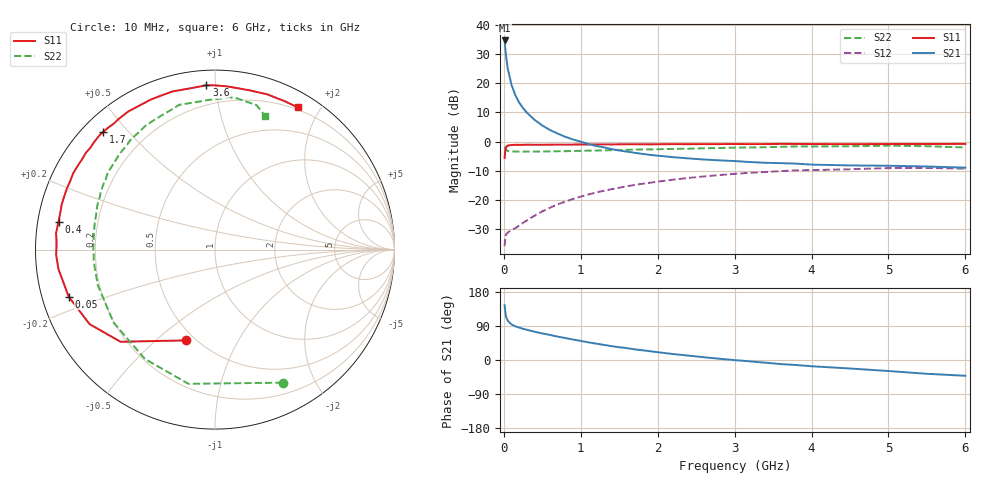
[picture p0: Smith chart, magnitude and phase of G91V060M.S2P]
! SIEMENS Small Signal Semiconductors
! BFG235
! Si NPN RF Bipolar Junction Transistor in SOT223
! VCE = 1 V  IC = 60 mA
! Common Emitter S-Parameters:  July  1994
# GHz  S  MA  R  50
!  f  S11  S21  S12  S22
! GHz  MAG  ANG  MAG  ANG  MAG  ANG  MAG  ANG
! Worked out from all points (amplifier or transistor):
!   40 points, 10 MHz to 6 GHz, reference 50 ohm
!   highest |S21| = 34.6 dB at 10 MHz (marker M1)
!   |S21| within 3 dB of that: start of sweep to 20.02 MHz
!   unconditionally stable (mu >= 1): 458.4 MHz to 1.645 GHz; 1.765 GHz to 1.95 GHz
!   at 200 MHz: K = 0.73, MSG = 21.0 dB, |S12| = -28.6 dB
!   at 1.5 GHz: K = 1.02, MAG = 5.5 dB, |S12| = -15.7 dB
!   at 6 GHz: K = 0.96, MSG = 0.2 dB, |S12| = -9.2 dB
!   S11 on the Smith chart (normalised r, x): 10 MHz: 0.45, -0.63; 50 MHz: 0.08, -0.16; 400 MHz: 0.06, +0.09; 1.7 GHz: 0.06, +0.43; 3.6 GHz: 0.08, +0.95; 6 GHz: 0.17, +1.73
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0.01  0.5304 -107.5  53.68 144.5  0.0164 55.9  0.8313 -63.1
0.02  0.7352 -135.7  38.03 124.7  0.0235 38.8  0.7623 -101.2
0.03  0.8131 -149.3  28.2 113.9  0.0259 31.9  0.7235 -122.7
0.05  0.8565 -162.2  18 103.7  0.028 25.7  0.6962 -144.3
0.1  0.8788 -172.9  9.287 93.9  0.0309 27.7  0.6823 -163.2
0.15  0.8856 -178.1  6.21 88.8  0.0334 33.8  0.6772 -170.8
0.2  0.8833 178.9  4.641 85.4  0.037 38.2  0.678 -175.0
0.25  0.8849 176.4  3.739 82.2  0.0411 42.5  0.6767 -178.1
0.3  0.8903 174.1  3.131 79.7  0.0452 45.7  0.6784 179.4
0.4  0.8856 169.9  2.359 74.6  0.0545 49.8  0.6776 175.7
0.5  0.8862 166.3  1.89 70.1  0.0644 52.6  0.6806 172.6
0.6  0.8906 163.5  1.585 66.2  0.0744 53.7  0.683 169.8
0.7  0.8911 159.9  1.373 61.7  0.0849 54.3  0.6871 167.1
0.9  0.8926 154.4  1.091 54.0  0.1052 53.0  0.6933 162.4
1.1  0.8959 148.1  0.912 46.5  0.1254 51.0  0.7036 157.7
1.7  0.9052 133.4  0.646 28.1  0.1825 41.7  0.7322 145.2
2.2  0.9088 122.1  0.544 15.7  0.2242 32.7  0.7532 134.9
3.2  0.909 100.9  0.449 -3.6  0.2938 13.6  0.7965 115.6
3.6  0.9169 93.0  0.43 -10.7  0.3143 5.2  0.8164 107.3
4.5  0.908 78.0  0.393 -22.4  0.3386 -10.3  0.8362 91.5
5.5  0.9132 65.1  0.377 -36.4  0.3561 -27.8  0.8375 74.0
6  0.9172 59.7  0.36 -41.6  0.3455 -34.4  0.7965 69.5
